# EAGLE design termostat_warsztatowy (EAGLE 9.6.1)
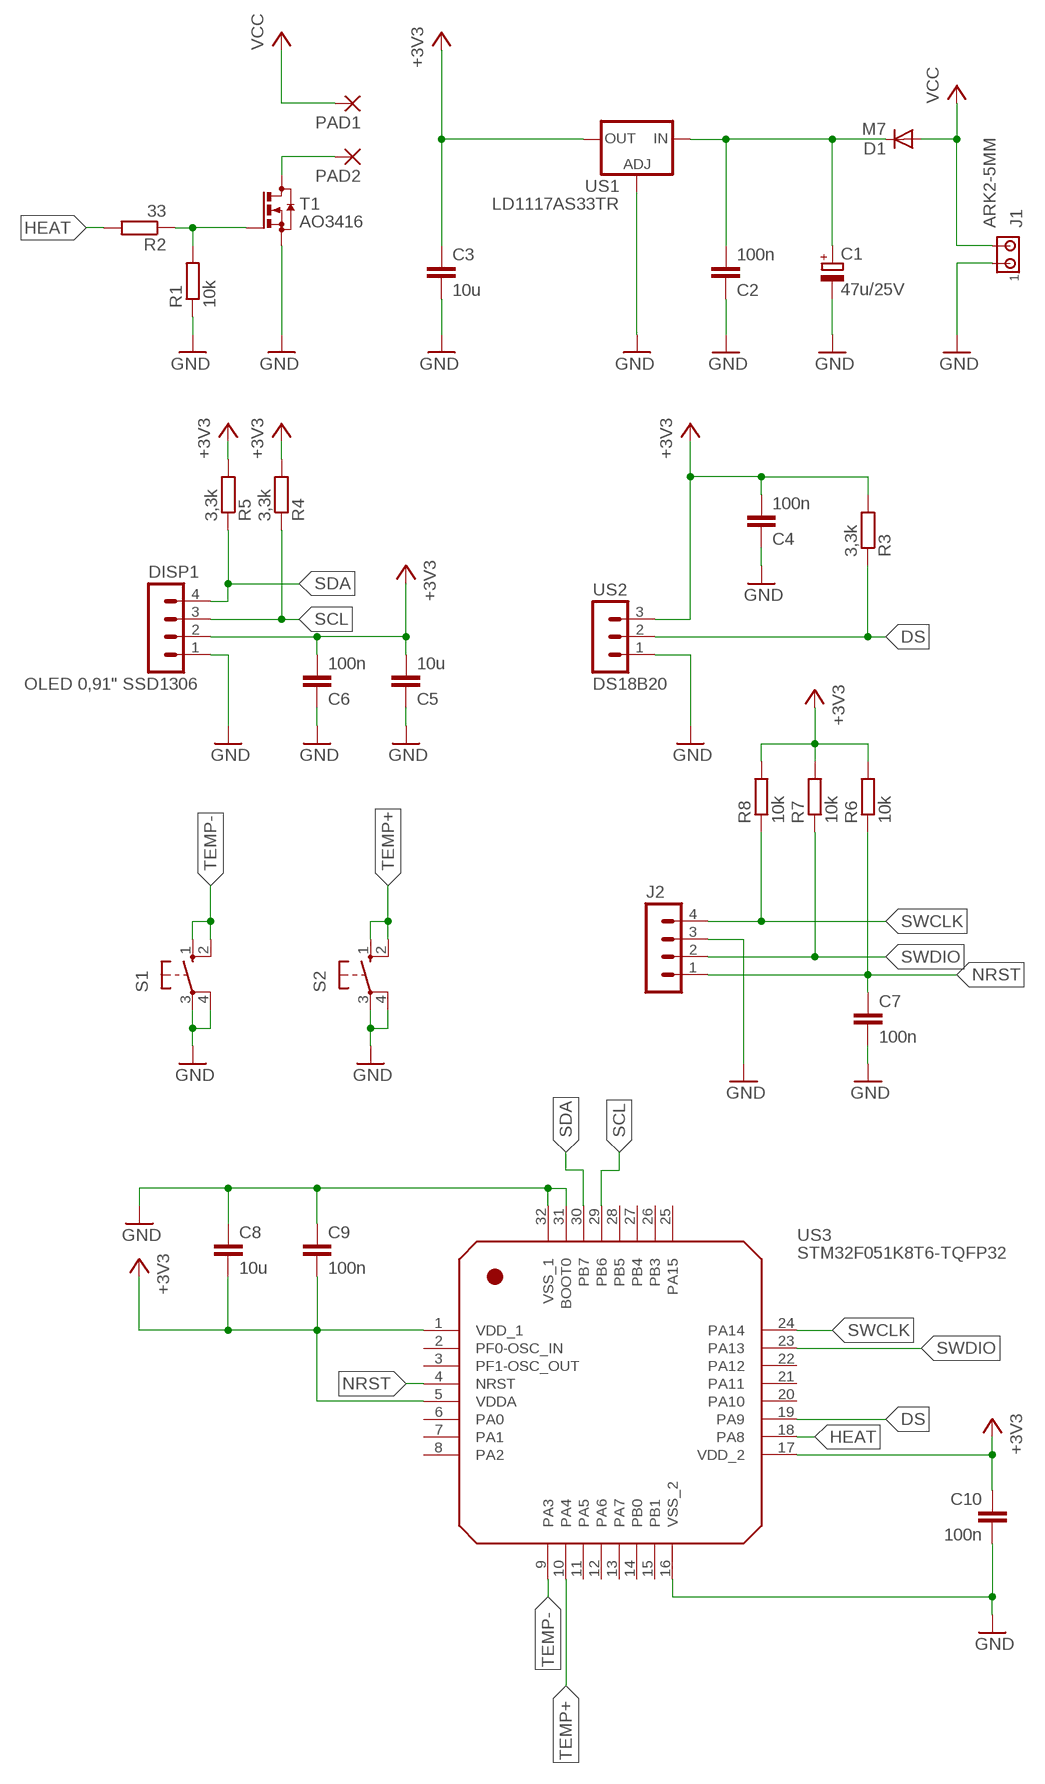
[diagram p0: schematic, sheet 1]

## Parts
C1  47u/25V  CPOL-EUE2.5-5  [E2,5-5]
C2  100n  C-EUC0805  [C0805]
C3  10u  C-EUC0805  [C0805]
C4  100n  C-EUC0805  [C0805]
C5  10u  C-EUC0805  [C0805]
C6  100n  C-EUC0805  [C0805]
C7  100n  C-EUC0805  [C0805]
C8  10u  C-EUC0805  [C0805]
C9  100n  C-EUC0805  [C0805]
C10  100n  C-EUC0805  [C0805]
D1  M7  DIODE-DO-214AC  [DO-214AC]
DISP1  OLED 0,91" SSD1306  MA04-1  [MA04-1]
J1  ARK2-5MM  ARK2-5MM-WASKI  [2PIN-5MM-WASKI]
J2  MA04-1  [MA04-1]
PAD1  2,54/0,8  [2,54/0,8]
PAD2  2,54/0,8  [2,54/0,8]
R1  10k  R-EU_R0805  [R0805]
R2  33  R-EU_R0805  [R0805]
R3  3,3k  R-EU_R0805  [R0805]
R4  3,3k  R-EU_R0805  [R0805]
R5  3,3k  R-EU_R0805  [R0805]
R6  10k  R-EU_R0805  [R0805]
R7  10k  R-EU_R0805  [R0805]
R8  10k  R-EU_R0805  [R0805]
S1  10-XX  [B3F-10XX]
S2  10-XX  [B3F-10XX]
T1  AO3416  BSS123  [SOT23]
US1  LD1117AS33TR  LD117AS33TR  [SOT223]
US2  DS18B20  MA03-1  [MA03-1]
US3  STM32F051K8T6-TQFP32  STM32F051-TQFP32  [TQFP32]

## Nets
+3V3: C3.1 C4.2 C5.2 C6.2 C8.2 C9.2 C10.1 DISP1.2 R3.2 R4.2 R5.2 R6.2 R7.2 R8.2 US1.4(OUT) US2.3 US3.1(VDD_1) US3.5(VDDA) US3.17(VDD_2)
DS: R3.1 US2.2 US3.19(PA9)
GND: C1.- C2.1 C3.2 C4.1 C5.1 C6.1 C7.2 C8.1 C9.1 C10.2 DISP1.1 J1.P$1 J2.3 R1.1 S1.3(P) S1.4(P1) S2.3(P) S2.4(P1) T1.2(S) US1.1(ADJ) US2.1 US3.16(VSS_2) US3.31(BOOT0) US3.32(VSS_1)
HEAT: R2.2 US3.18(PA8)
N$1: C1.+ C2.2 D1.C US1.3(IN)
N$2: PAD2.1(P) T1.3(D)
N$3: R1.2 R2.1 T1.1(G)
NRST: C7.1 J2.1 R6.1 US3.4(NRST)
SCL: DISP1.3 R4.1 US3.29(PB6)
SDA: DISP1.4 R5.1 US3.30(PB7)
SWCLK: J2.4 R8.1 US3.24(PA14)
SWDIO: J2.2 R7.1 US3.23(PA13)
TEMP+: S2.1(S) S2.2(S1) US3.10(PA4)
TEMP-: S1.1(S) S1.2(S1) US3.9(PA3)
VCC: D1.A J1.P$2 PAD1.1(P)
Unconnected: US3.2(PF0-OSC_IN) US3.3(PF1-OSC_OUT) US3.6(PA0) US3.7(PA1) US3.8(PA2) US3.11(PA5) US3.12(PA6) US3.13(PA7) US3.14(PB0) US3.15(PB1) US3.20(PA10) US3.21(PA11) US3.22(PA12) US3.25(PA15) US3.26(PB3) US3.27(PB4) US3.28(PB5)

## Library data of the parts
C1 = rcl:CPOL-EU: POLARIZED CAPACITOR, European symbol
C2-C10 = rcl:C-EU: CAPACITOR, European symbol
D1 = diode:DIODE-: DIODE
DISP1 J2 = con-lstb:MA04-1: PIN HEADER; OC_FARNELL: unknown; OC_NEWARK: unknown
J1 = zlacza_futrzak:ARK2: ARK 2
PAD1 PAD2 = wirepad:2,54/0,8: THROUGH-HOLE PAD
R1-R8 = rcl:R-EU_: RESISTOR, European symbol
S1 S2 = switch-omron:10-XX: OMRON SWITCH; MPN: B3F-1000; OC_FARNELL: 176432; OC_NEWARK: 36M3542
T1 = transistor-small-signal:BSS123: N-CHANNEL MOS FET
US1 = v-reg:LD117A?*: Low drop fixed and adjustable positive voltage regulators 1 A Source: http://www.st.com/stonline/products/literature/ds/7194/ld1117axx.pdf
US2 = zlacza_futrzak:MA03-1: PIN HEADER; OC_FARNELL: unknown; OC_NEWARK: unknown
US3 = scalaki_futrzak:STM32F051-TQFP32

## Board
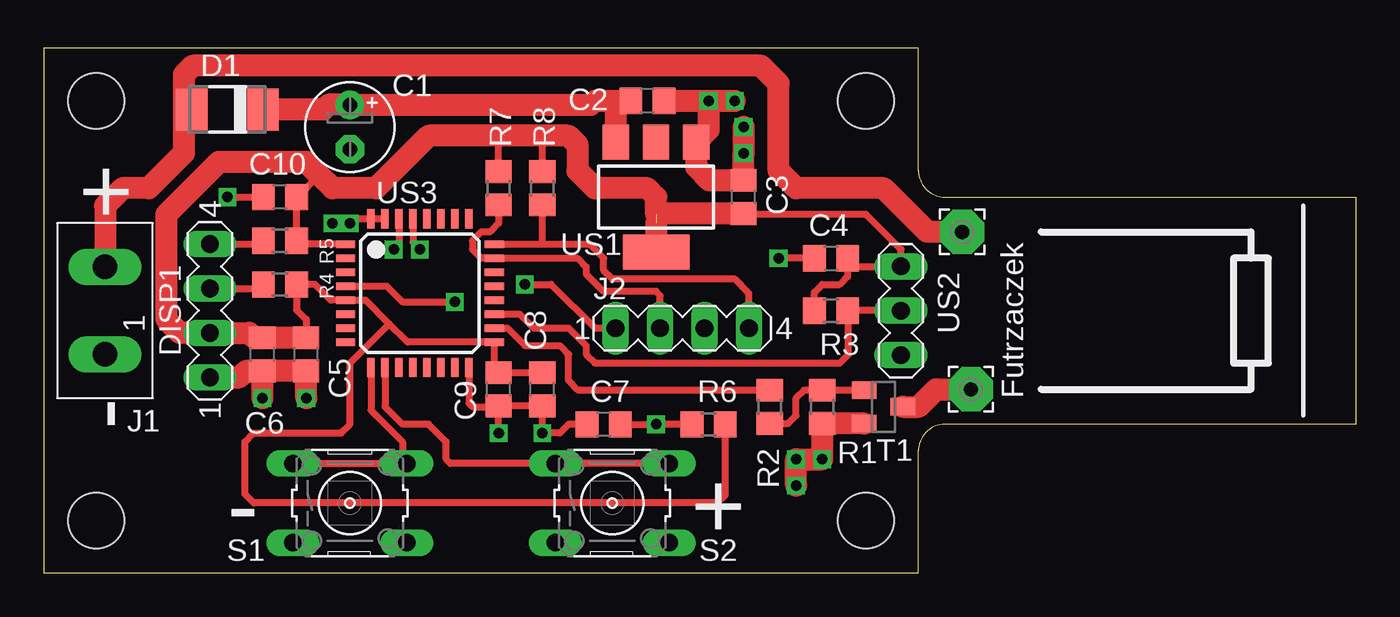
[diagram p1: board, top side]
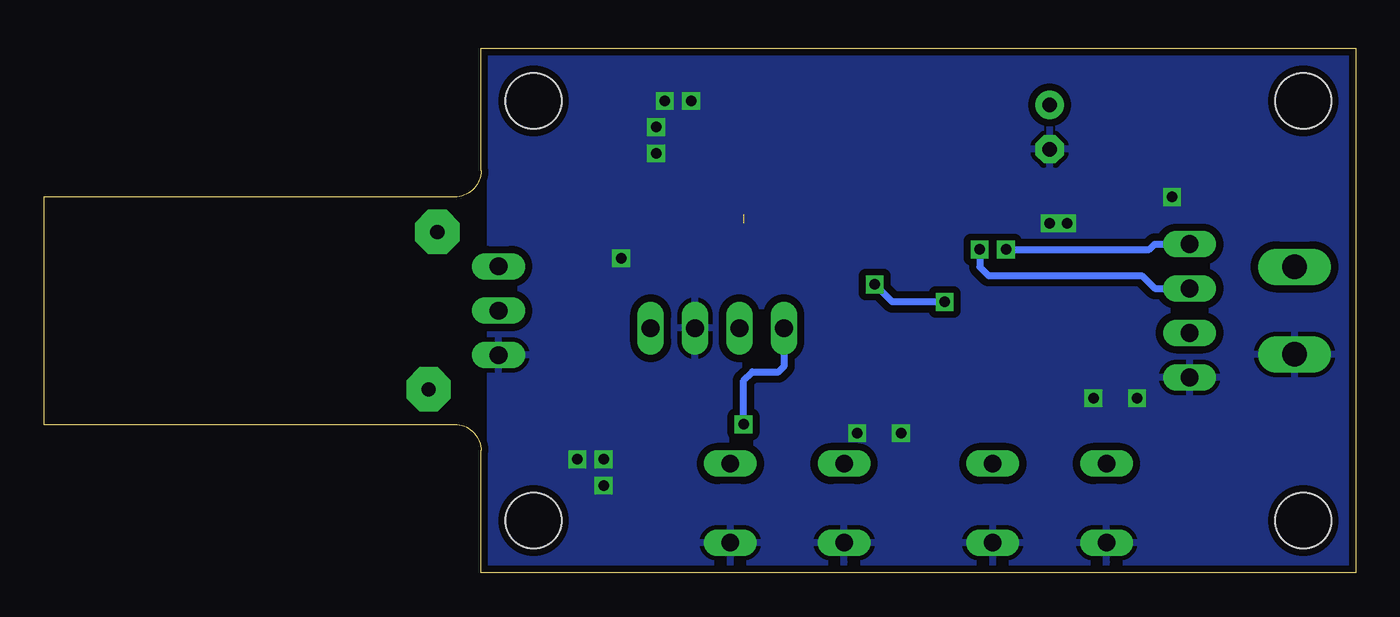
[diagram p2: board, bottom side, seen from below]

Size 75 x 30 mm. Coordinates in mm from the lower left corner, seen from the top.
Outline: 0,0 50,0 50,7 arc-90 51.5,8.5 75,8.5 75,21.5 51.5,21.5 arc-90 50,23 50,30 0,30 0,0
Copper layers (1*16): Top 0.035mm / dielectric 1.5mm / Bottom 0.035mm
Design rules: minimum track width 10mil, minimum drill 23mil, track to track 8mil, track to pad 8mil, pad to pad 8mil, via to via 8mil, smd to smd 8mil, copper to edge 10mil, drill to drill 8mil, minimum pad ring 10mil, minimum via ring 8mil, stop-mask expansion 4mil, vias tented up to drill 0mil, thermal gap 10mil
Holes 3.2 mm at 3,3 47,3 3,27 47,27

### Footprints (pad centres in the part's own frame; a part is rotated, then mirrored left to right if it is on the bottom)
E2,5-5 = drill 0.813 pad 1.6: + -1.27,0 | drill 0.813 pad 1.6 octagon: - 1.27,0
C0805 = smd 1.3 x 1.5: 1 -0.95,0; 2 0.95,0
DO-214AC = smd 1.8 x 2.4: A 2.025,0; C -2.025,0
MA04-1 = drill 1.016 long: 1 -3.81,0; 2 -1.27,0; 3 1.27,0; 4 3.81,0
2PIN-5MM-WASKI = drill 1.4 long: P$1 -2.5,0; P$2 2.5,0
2,54/0,8 = drill 0.813 pad 2.54 octagon: 1 0,0
R0805 = smd 1.3 x 1.5: 1 -0.95,0; 2 0.95,0
B3F-10XX = drill 1.016 long: 1 -3.251,2.261; 2 3.251,2.261; 3 -3.251,-2.261; 4 3.251,-2.261
SOT23 = smd 1 x 1.4: 1 -0.95,-1.1; 2 0.95,-1.1; 3 0,1.1
SOT223 = smd 1.5 x 2: 1 -2.3,-3.15; 2 0,-3.15; 3 2.3,-3.15 | smd 3.8 x 2: 4 0,3.15
MA03-1 = drill 1.016 long: 1 -2.54,0; 2 0,0; 3 2.54,0
TQFP32 = smd 1.1 x 0.45: 1 -4.25,2.8; 2 -4.25,2; 3 -4.25,1.2; 4 -4.25,0.4; 5 -4.25,-0.4; 6 -4.25,-1.2; 7 -4.25,-2; 8 -4.25,-2.8; 17 4.25,-2.8; 18 4.25,-2; 19 4.25,-1.2; 20 4.25,-0.4; 21 4.25,0.4; 22 4.25,1.2; 23 4.25,2; 24 4.25,2.8 | smd 0.45 x 1.1: 9 -2.8,-4.25; 10 -2,-4.25; 11 -1.2,-4.25; 12 -0.4,-4.25; 13 0.4,-4.25; 14 1.2,-4.25; 15 2,-4.25; 16 2.8,-4.25; 25 2.8,4.25; 26 2,4.25; 27 1.2,4.25; 28 0.4,4.25; 29 -0.4,4.25; 30 -1.2,4.25; 31 -2,4.25; 32 -2.8,4.25

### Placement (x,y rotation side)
C1  17.5,25.5 270 top
C2  34.5,27 180 top
C3  40,21.5 90 top
C4  45,18 0 top
C5  15,12.5 90 top
C6  12.5,12.5 90 top
C7  32,8.5 180 top
C8  28.5,10.5 90 top
C9  26,10.5 90 top
C10  13.5,21.5 180 top
D1  10.5,26.5 180 top
DISP1  9.5,15 90 top
J1  3.5,15 90 top
J2  36.5,14 0 top
PAD1  52.5,19.5 0 top
PAD2  53,10.5 0 top
R1  44.5,9.5 90 top
R2  41.5,9.5 90 top
R3  45,15 180 top
R4  13.5,16.5 0 top
R5  13.5,19 0 top
R6  38,8.5 0 top
R7  26,22 90 top
R8  28.5,22 90 top
S1  17.5,4 0 top
S2  32.5,4 0 top
T1  48,9.5 270 top
US1  35,21.5 180 top
US2  49,15 90 top
US3  21.5,16 0 top

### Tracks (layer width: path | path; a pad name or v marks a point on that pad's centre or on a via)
+3V3  (1 unrouted)
  Top 0.406: C3.1 40.05,20.5 47,20.5 49,18.5 US2.3 48.96,17.5 46.45,17.5 C4.2 45.95,16.95 45.5,16.5 44.5,16.5 44.05,16.05 R3.2 | C5.2 15,14.5 14.45,15.05 R4.2 15.5,16.5 16.4,15.6 US3.5 18.4,15.6 19.75,14.25 | US3.1 14.75,18.8 14.45,18.5 R5.2 C10.1 14.5,21.5 15.75,22.75 | 19.75,14.25 20.8,13.2 US3.17 25.75,11.7 C9.2 C8.2 | R8.2 28.5,25 | R7.2 26,25 | R6.2 38.95,4.45 38.5,4 12,4 11.5,4.5 11.5,7.5 12,8 17,8 17.5,8.5 17.5,12 19.75,14.25
  Top 1.27: C3.1 35.05,20.55 35,20.5 35,21.5 34.5,22 31.5,22 30.5,23 30.5,24.5 30,25 28.5,25 26,25 22,25 19,22 16.5,22 15.75,22.75 15,23.5 10,23.5 7,20.5 7,14.5 7.77,13.73 DISP1.2 11.77,13.73 12.05,13.45 C6.2 C5.2 | 35,20 US1.4
DS
  Top 0.406: US2.2 R3.1 46,14.95 46,12.5 45.5,12 31.5,12 31,12.5 31,13 30,14 28,14 27.2,14.8 US3.19
GND  (via drill 0.6)
  Top 0.406: C4.1 v42,18 | v10.5,21.5 C10.2 | US3.31 US3.32 17.75,20.25 v17.5,20 v16.5,20 | v26,8 C9.1 | C9.1 C8.1 v28.5,8 29.5,8 30,8.5 C7.2 | US3.16 24.3,9.7 24.5,9.5 25.95,9.5 C9.1
  Top 1.27: C2.1 v38,27 | v38,27 v39.5,27 | v40,25.5 v40,24 C3.2 38.05,22.45 37.3,23.2 US1.1 38,25.35 v38,27 | v15,10 C5.1 C6.1 | v12.5,10 C6.1 | C6.1 11.55,11.55 11.19,11.19 DISP1.1 | v43,5 v43,6.5 v44.5,6.5 R1.1 T1.2
  pour Bottom (isolate 0.406): 0,30 49.5,30 49.5,0 0,0
HEAT
  Top 0.406: US3.18 26.5,14 27.5,13 29.5,13 30,12.5 30,11 30.55,10.45 R2.2
N$1
  Top 1.27: D1.C 16,26.5 16.27,26.77 C1.+ 31.27,26.77 31.5,27 32.5,27 | 32.5,27 C2.2 | US1.3 32.7,26.8 32.5,27
N$2
  Top 1.27: T1.3 50,9.5 51,10.5 PAD2.1
N$3
  Top 0.406: T1.1 R1.2 43.45,10.45 43,10 43,9 42.55,8.55 R2.1
NRST  (via drill 0.6)
  Top 0.406: US3.4 19.6,16.4 20.5,15.5 v23.5,15.5 | C7.1 v35,8.5 R6.1 | v27.5,16.5 29,16.5 31.5,14 J2.1
  Bottom 0.406: v23.5,15.5 26.5,15.5 v27.5,16.5 | v35,8.5 35,11 34.5,11.5 33,11.5 32.69,11.81 J2.1
SCL  (via drill 0.6)
  Top 0.406: DISP1.3 12.32,16.27 R4.1 | v21.5,18.5 21.1,18.9 US3.29
  Bottom 0.406: v21.5,18.5 21.5,17.5 21,17 12.23,17 11.5,16.27 DISP1.3
SDA  (via drill 0.6)
  Top 0.406: DISP1.4 12.36,18.81 R5.1 | US3.30 20.3,18.8 v20,18.5
  Bottom 0.406: v20,18.5 11.81,18.5 11.5,18.81 DISP1.4
SWCLK
  Top 0.406: 28.5,18.8 R8.1 | J2.4 40.31,15.99 39.5,16.8 32.5,16.8 32,17.3 32,18 31.2,18.8 28.5,18.8 | US3.24 28.5,18.8
SWDIO
  Top 0.406: R7.1 26,20 25.5,19.5 25,19.5 24.5,19 24.5,18.5 25,18 US3.23 30.5,18 31,17.5 31,17.1 32,16.1 35,16.1 35.23,15.87 J2.2
TEMP+
  Top 0.406: S2.2 S2.1 23.24,6.26 23,6.5 23,7.5 22,8.5 20.5,8.5 19.5,9.5 US3.10
TEMP-
  Top 0.406: US3.9 18.7,9.3 20.5,7.5 20.5,6.51 S1.2 S1.1
VCC
  Top 1.27: PAD1.1 50.5,19.5 48,22 43,22 42,23 42,28 41,29 8.5,29 8,28.5 8,26.5 | 8,26.5 8,24 6,22 4.5,22 3.5,21 J1.P$2 | D1.A 8,26.5

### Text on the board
tPlace: + | - | Futrzaczek | - | +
